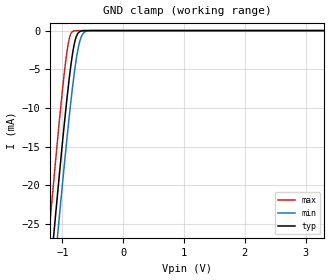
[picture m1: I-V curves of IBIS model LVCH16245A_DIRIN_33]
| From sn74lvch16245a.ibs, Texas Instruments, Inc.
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[Model]   LVCH16245A_DIRIN_33
Model_type  Input
Vinl=0.8
Vinh=2.0
| variable   typ   min   max
C_comp   2.75pF   2.12pF   3.61pF
[Temperature Range]   40   100   -40
| Ambient temperature   25   85   -40
[Voltage range]   3.3   3   3.6
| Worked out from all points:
|   GND clamp passes 1 mA (typ) near -0.78 V on its own axis
[GND Clamp]
| LVCH16245A_DIRIN_33
|   Voltage   I(typ)   I(min)   I(max)
-5V       -385.1mA   -389.7mA   -379.3mA
-1.215V   -32.71mA   -38.18mA   -25.7mA
-1.14V    -26.2mA    -31.67mA   -19.18mA
-1.08V    -21.09mA   -26.54mA   -14.1mA
-1.06V    -19.42mA   -24.86mA   -12.46mA
-925mV    -8.768mA   -13.92mA   -2.718mA
-875mV    -5.359mA   -10.19mA   -702.5uA
-820mV    -2.36mA    -6.447mA   -72.13uA
-770mV    -743.6uA   -3.591mA   -7.079uA
-715mV    -135.5uA   -1.404mA   -533.3nA
-590mV    -1.781uA   -53.99uA   -1.489nA
3.3V      6.303pA    8.434pA    5.93pA
